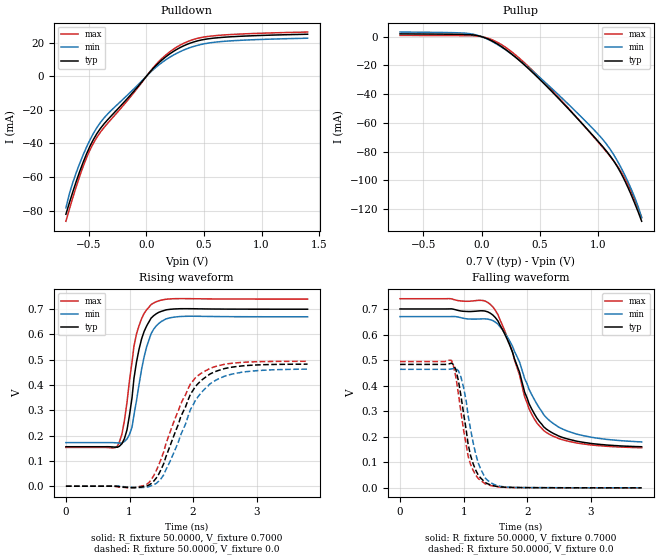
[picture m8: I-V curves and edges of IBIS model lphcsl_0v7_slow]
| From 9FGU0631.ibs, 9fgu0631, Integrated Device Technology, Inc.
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[Model]  lphcsl_0v7_slow
Model_type Output
Polarity   Non-Inverting
Enable   Active-High
Vmeas =  0.4000V
Cref =   2.0000pF
Rref =   0.0
Vref =   0.4000V
C_comp   1.1000pF   1.0000pF   1.2000pF
[Temperature Range]   25.0000   75.0000   0.0
[Voltage Range]   0.7000V   0.6700V   0.7400V
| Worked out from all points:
|   slope of the pulldown table from 0 to 0.105 V, typ, clamps not added: 13.4 ohm
|   slope of the pullup table from 0 to 0.105 V, typ, clamps not added: 28.5 ohm
|   rising waveform, R_fixture 50.0000, V_fixture 0.7000: 20-80 % time 213ps typ, 231ps min, 209ps max; typ from 0.156 V to 0.7 V
|   rising waveform, R_fixture 50.0000, V_fixture 0.0: 20-80 % time 468ps typ, 505ps min, 457ps max; typ from 0 V to 0.483 V
|   falling waveform, R_fixture 50.0000, V_fixture 0.7000: 20-80 % time 500ps typ, 559ps min, 471ps max; typ from 0.7 V to 0.161 V
|   falling waveform, R_fixture 50.0000, V_fixture 0.0: 20-80 % time 206ps typ, 221ps min, 199ps max; typ from 0.483 V to 0 V
[Pulldown]
|Voltage   I(typ)   I(min)   I(max)
-700mV    -82.14mA   -78.33mA   -86.3mA
-640mV    -68.79mA   -63.21mA   -72.24mA
-580mV    -56.64mA   -51.82mA   -59.42mA
-490mV    -41.54mA   -37.77mA   -43.75mA
-430mV    -34.05mA   -30.48mA   -36.23mA
-340mV    -26.12mA   -22.67mA   -28.22mA
-130mV    -10.53mA   -8.891mA   -11.53mA
20mV      1.656mA    1.382mA    1.825mA
200mV     13.17mA    11.18mA    14.37mA
350mV     18.87mA    16.29mA    20.4mA
530mV     22.18mA    19.61mA    23.61mA
1.4V      24.97mA    22.6mA     26.27mA
[Pullup]
|Voltage   I(typ)   I(min)   I(max)
-700mV    1.953mA    3.23mA     886.9uA
-70mV     1.182mA    1.633mA    602.4uA
80mV      -2.622mA   -2.943mA   -1.863mA
230mV     -10.45mA   -10.65mA   -8.914mA
350mV     -18.55mA   -18.18mA   -17.01mA
530mV     -32.42mA   -30.85mA   -31.3mA
830mV     -57.91mA   -54.07mA   -57.81mA
1.04V     -76.91mA   -71.94mA   -77.46mA
1.13V     -86.5mA    -82.16mA   -86.47mA
1.22V     -99.41mA   -95.52mA   -97.83mA
1.31V     -116mA     -111.9mA   -113.4mA
1.37V     -128.6mA   -126.2mA   -125.8mA
[Ramp]
| variable   typ   min   max
dV/dt_r  0.2896/0.5041n   0.2778/0.5371n   0.2965/0.4799n
dV/dt_f  0.3235/0.5324n   0.2941/0.5976n   0.3499/0.5046n
R_load = 50.0000
[Rising Waveform]
R_fixture= 50.0000
V_fixture= 0.7000
V_fixture_min= 0.6700
V_fixture_max= 0.7400
|time   V(typ)   V(min)   V(max)
0s        156.1mV    172.3mV    153.3mV
810ps     154.1mV    171.1mV    158.4mV
880ps     167.7mV    170.6mV    205.2mV
960ps     222.1mV    186.9mV    330.9mV
1.04ns    350.5mV    233.8mV    491.8mV
1.11ns    491.2mV    338.5mV    602.3mV
1.23ns    612.1mV    511.7mV    683.5mV
1.38ns    674.3mV    621.1mV    724.6mV
1.77ns    701.6mV    670.5mV    741.8mV
3.8ns     700mV      670mV      740mV
[Rising Waveform]
R_fixture= 50.0000
V_fixture= 0.0
V_fixture_min= 0.0
V_fixture_max= 0.0
|time   V(typ)   V(min)   V(max)
0s        0V         0V         0V
1ns       -5.064mV   -3.942mV   -6.457mV
1.31ns    5.075mV    -1.264mV   15.36mV
1.42ns    32mV       10.98mV    61.28mV
1.54ns    90.43mV    45.69mV    137.4mV
1.8ns     270.5mV    199.7mV    322.1mV
1.96ns    365mV      304.1mV    405.4mV
2.26ns    442.9mV    403.4mV    465.3mV
2.76ns    475.5mV    450.5mV    489.6mV
3.8ns     482.7mV    463mV      494.1mV
[Falling Waveform]
R_fixture= 50.0000
V_fixture= 0.7000
V_fixture_min= 0.6700
V_fixture_max= 0.7400
|time   V(typ)   V(min)   V(max)
0s        700mV      670mV      740mV
1.38ns    688.6mV    660.2mV    725.5mV
1.54ns    653.1mV    640.5mV    677.9mV
1.69ns    578.6mV    589.5mV    586.6mV
1.88ns    452.1mV    492.2mV    441.1mV
1.96ns    374.4mV    427.4mV    356.3mV
2.03ns    328.8mV    385.4mV    308.8mV
2.26ns    238.7mV    286.2mV    224mV
2.76ns    183.5mV    211.5mV    176.3mV
3.8ns     160.8mV    179.8mV    156.9mV
[Falling Waveform]
R_fixture= 50.0000
V_fixture= 0.0
V_fixture_min= 0.0
V_fixture_max= 0.0
|time   V(typ)   V(min)   V(max)
0s        483mV      463.8mV    494.2mV
810ps     487.9mV    465.1mV    498.4mV
880ps     461.7mV    466.4mV    431.4mV
960ps     357.8mV    432.4mV    293.9mV
1.04ns    228.1mV    341.3mV    170.9mV
1.07ns    172.6mV    285.3mV    125.1mV
1.19ns    69.42mV    132.8mV    50.16mV
1.34ns    20.93mV    38.52mV    15.76mV
1.69ns    2.025mV    2.898mV    1.619mV
3.8ns     64.13uV    98.46uV    50.29uV
